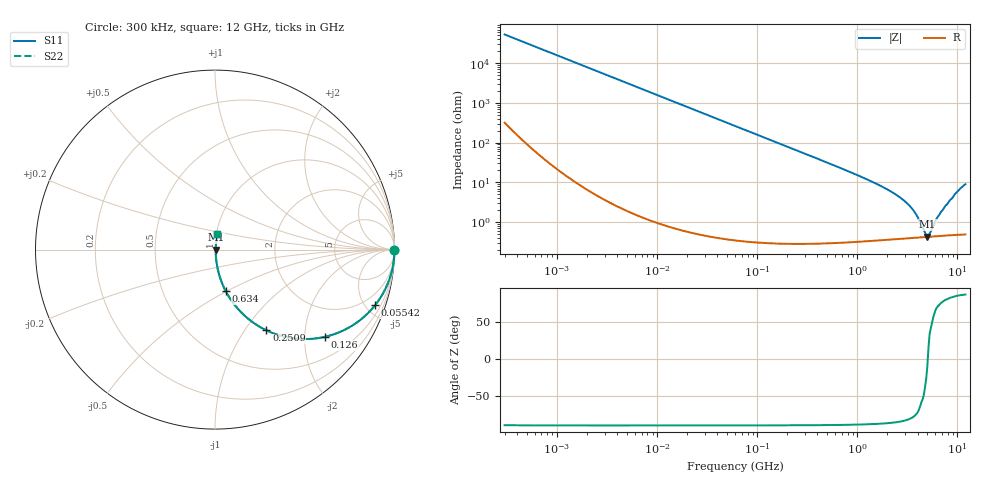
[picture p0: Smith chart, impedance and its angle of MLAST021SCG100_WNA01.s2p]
! MLAST021SCG100_WNA01  S-PARAMETER MODEL  ( General Type )
! Model Generated by TAIYO YUDEN Corporation (http://www.ty-top.com)
! Version 1.0
! TAIYO YUDEN Control No. 220901
! Copyright(c) 2022 TAIYO YUDEN CO.,LTD. All Rights Reserved.
! Product Description (link to TY-COMPAS)
! https://ds.yuden.co.jp/TYCOMPAS/or/detail?pn=MLAST021SCG100CWNA01&u=M
! Products Name : Multilayer Ceramic Capacitors
! Characteristics :
!  Capacitance : 10 pF , Rated Voltage : 25V , TCC : CG / C0G
!  Case Size : 0.25 x 0.125 / 0.0098 x 0.0049 [mm/inch] , Thickness : 0.125 / 0.0049 [mm/inch]
!  (Conditions: Temperature = 25 degC , DC Bias Current/Voltage = 0A / 0V)
! External Node Assignments :
!  1  o---| |---o  2
! GND o---------o GND
! Frequency Range : 0.3MHz  -  12000MHz  [ 401 STEP ]
# MHz S RI R 50
! Freq[MHz].  S11 Real  S11 Imag  S21 Real  S21 Imag  S12 Real  S12 Imag  S22 Real  S22 Imag
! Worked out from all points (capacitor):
!   401 points, 300 kHz to 12 GHz, reference 50 ohm
!   read as one part in series: C = 10 pF near 316.3 kHz
!   lowest |Z| = 432 mohm at 5.006 GHz (marker M1)
!   series resonance near 5.055 GHz, so ESL is about 99 pH
!   S11 on the Smith chart (normalised r, x): 300 kHz: open; 55.42 MHz: 1.01, -5.74; 126 MHz: 1.01, -2.53; 250.9 MHz: 1.01, -1.27; 634 MHz: 1.01, -0.49; 12 GHz: 1.01, +0.18
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0.3  1 -0.00188  1.48e-05 0.00188  1.48e-05 0.00188  1 -0.00188
1.769972  0.9999 -0.0111  0.000133 0.0111  0.000133 0.0111  0.9999 -0.0111
10.44266  0.9957 -0.0653  0.00433 0.0653  0.00433 0.0653  0.9957 -0.0653
25.03118  0.9757 -0.1534  0.0243 0.1534  0.0243 0.1534  0.9757 -0.1534
55.41608  0.8915 -0.3103  0.1085 0.3103  0.1085 0.3103  0.8915 -0.3103
60  0.8752 -0.3298  0.1248 0.3298  0.1248 0.3298  0.8752 -0.3298
125.9782  0.6142 -0.4856  0.3858 0.4856  0.3858 0.4856  0.6142 -0.4856
177.7716  0.4444 -0.4953  0.5556 0.4953  0.5556 0.4953  0.4444 -0.4953
250.8588  0.2868 -0.45  0.7132 0.45  0.7132 0.45  0.2868 -0.45
353.9943  0.1682 -0.3709  0.8318 0.3709  0.8318 0.3709  0.1682 -0.3709
634.0297  0.0599 -0.2313  0.9401 0.2313  0.9401 0.2313  0.0599 -0.2313
2088.533  0.0074 -0.0614  0.9926 0.0614  0.9926 0.0614  0.0074 -0.0614
2795.104  0.00524 -0.0377  0.9948 0.0377  0.9948 0.0377  0.00524 -0.0377
3454.93  0.00448 -0.0226  0.9955 0.0226  0.9955 0.0226  0.00448 -0.0226
3841.137  0.00428 -0.0154  0.9957 0.0154  0.9957 0.0154  0.00428 -0.0154
4747.894  0.00422 -0.00327  0.9958 0.00327  0.9958 0.00327  0.00422 -0.00327
5006.236  0.00425 -0.000707  0.9958 0.000707  0.9958 0.000707  0.00425 -0.000707
5278.635  0.0043 0.00289  0.9957 -0.00289  0.9957 -0.00289  0.0043 0.00289
6354.153  0.00459 0.0127  0.9954 -0.0127  0.9954 -0.0127  0.00459 0.0127
7254.098  0.00497 0.021  0.995 -0.021  0.995 -0.021  0.00497 0.021
9968.853  0.00808 0.0575  0.9919 -0.0575  0.9919 -0.0575  0.00808 0.0575
12000  0.0128 0.0884  0.9872 -0.0884  0.9872 -0.0884  0.0128 0.0884
